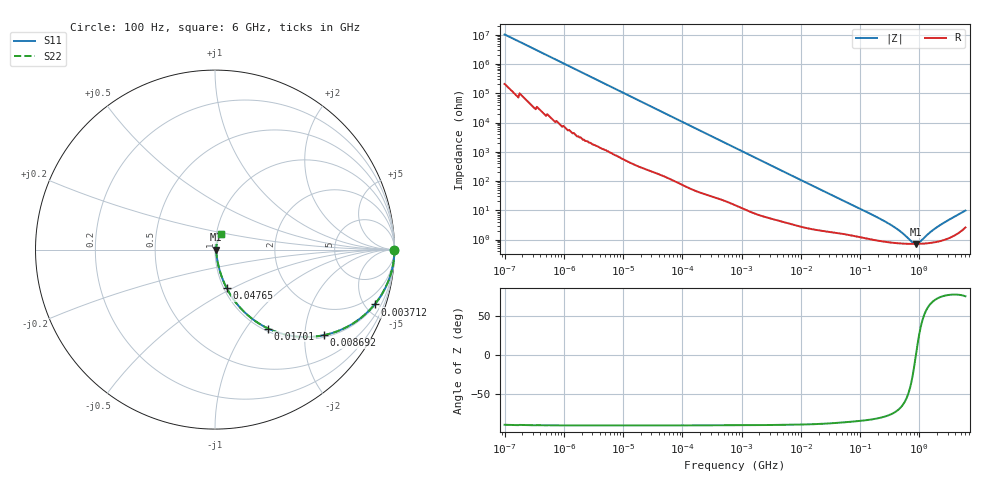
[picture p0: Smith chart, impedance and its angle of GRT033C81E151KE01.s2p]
!Murata Part Number: GRT033C81E151KE01
!These Parameters are Measured in Series Mode Connection
!Data Generated on Jun 19, 2026
!  o--ll--o
!Port1  Port2
!  o------o
!Operation Temp=25[degC], DC Bias Voltage=0[V]
!Freq. Start=100[Hz] Stop=6[GHz] 401[Steps]
# Hz S RI R 50
!Freq.(Hz) S11(Real) S11(Imag) S21(Real) S21(Imag) S12(Real) S12(Imag) S22(Real) S22(Imag)
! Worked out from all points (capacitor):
!   401 points, 100 Hz to 6 GHz, reference 50 ohm
!   read as one part in series: C = 155 pF near 109 Hz
!   lowest |Z| = 710 mohm at 875 MHz (marker M1)
!   series resonance near 877.7 MHz, so ESL is about 210 pH
!   S11 on the Smith chart (normalised r, x): 100 Hz: open; 3.712 MHz: 1.09, -5.78; 8.692 MHz: 1.06, -2.49; 17.01 MHz: 1.04, -1.28; 47.65 MHz: 1.03, -0.46; 6 GHz: 1.05, +0.19
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100  1 -9.8e-06  2e-07 9.8e-06  2e-07 9.8e-06  1 -9.8e-06
981  1 -9.48e-05  7e-07 9.48e-05  7e-07 9.48e-05  1 -9.48e-05
2008  1 -0.000194  1.1e-06 0.000194  1.1e-06 0.000194  1 -0.000194
40335  1 -0.00385  4.01e-05 0.00385  4.01e-05 0.00385  1 -0.00385
774597  0.9939 -0.0724  0.00607 0.0724  0.00607 0.0724  0.9939 -0.0724
1734173  0.9725 -0.1576  0.0275 0.1576  0.0275 0.1576  0.9725 -0.1576
3712478  0.8891 -0.3059  0.1109 0.3059  0.1109 0.3059  0.8891 -0.3059
5554849  0.7853 -0.4009  0.2147 0.4009  0.2147 0.4009  0.7853 -0.4009
8692127  0.6052 -0.477  0.3948 0.477  0.3948 0.477  0.6052 -0.477
1.555665e7  0.3333 -0.4556  0.6667 0.4556  0.6667 0.4556  0.3333 -0.4556
1.701401e7  0.2967 -0.4401  0.7033 0.4401  0.7033 0.4401  0.2967 -0.4401
2.784235e7  0.1456 -0.3296  0.8544 0.3296  0.8544 0.3296  0.1456 -0.3296
4.764863e7  0.0646 -0.2137  0.9354 0.2137  0.9354 0.2137  0.0646 -0.2137
1.066761e8  0.0222 -0.1019  0.9778 0.1019  0.9778 0.1019  0.0222 -0.1019
3.124326e8  0.00903 -0.0326  0.991 0.0326  0.991 0.0326  0.00903 -0.0326
4.888888e8  0.00757 -0.0167  0.9924 0.0167  0.9924 0.0167  0.00757 -0.0167
7.650043e8  0.00706 -0.00373  0.9929 0.00373  0.9929 0.00373  0.00706 -0.00373
8.749838e8  0.00705 -8.09e-05  0.9929 8.09e-05  0.9929 8.09e-05  0.00705 -8.09e-05
1.000774e9  0.00712 0.00358  0.9929 -0.00358  0.9929 -0.00358  0.00712 0.00358
1.497423e9  0.00779 0.0152  0.9922 -0.0152  0.9922 -0.0152  0.00779 0.0152
2.142435e9  0.00933 0.0276  0.9907 -0.0276  0.9907 -0.0276  0.00933 0.0276
6e9  0.0334 0.089  0.9666 -0.089  0.9666 -0.089  0.0334 0.089
